| Integrated Devices Technolgy, Inc.
| IBIS Model Of 82P2821
| BH_640
[IBIS ver]	3.2
[File name]	82p2821.ibs
[File Rev]	1.0
[Date]		Aug. 15, 2005
[Source]	Integrated Devices Technolgy, Inc.
[Notes]   1. Temperatures: typ=25C, min=90C, max=-40C .
   2. simulator: hspice
   3. The IBIS models are validated with hspice models
[Disclaimer]	 Integrated Device Technology, Inc. ("IDT") hereby grants
		 the user of this IBIS model a non-exclusive, nontransferable
		 license to use this IBIS model under the following terms.
		 The user is granted this license only to use the IBIS model
		 and is not granted rights to sell, copy (except as needed to
		 run the IBIS model), rent, lease or sub-license the IBIS model
		 in whole or in part, or in modified form to anyone. The User
		 may modify the IBIS model to suit its specific applications,
		 but rights to derivative works and such modifications shall
		 belong to IDT. This IBIS model is provided on an AS IS" basis
		 and IDT makes absolutely no warranty with respect to the
		 information contained herein. IDT DISCLAIMS AND CUSTOMER WAIVES
		 ALL WARRANTIES, EXPRESS AND IMPLIED, INCLUDING WARRANTIES
		 OF MERCHANTABILITY AND FITNESS FOR A PARTICULAR PURPOSE. THE
		 ENTIRE RISK AS TO QUALITY AND PERFORMANCE IS WITH THE USER ACCORDINGLY,
		 IN NO EVENT SHALL IDT BE LIABLE FOR ANY DIRECT OR
		 INDIRECT DAMAGES, WHETHER IN CONTRACT OR TORT, INCLUDING ANY
		 LOST PROFITS OR OTHER INCIDENTAL, CONSEQUENTIAL, EXEMPLARY, OR
		 PUNITIVE DAMAGES ARISING OUT OF THE USE OR APPLICATION OF THE
		 IBIS model. Further, IDT reserves the right to make changes
		 without notice to
[Copyright]	Copyright 2005, Integrated Devices Technolgy, Inc.,
   All Rights Reserved.
|   Component 82P2821
[Component]	82P2821
[Manufacturer]	Integrated Devices Technolgy, Inc.
[Package]
| variable   typ   min   max
R_pkg   0.3500   0.2100   0.5700
L_pkg   7.3400nH   3.9900nH   14.3900nH
C_pkg   0.8400pF   0.2900pF   2.2800pF
[Pin]  signal_name   model_name   R_pin   L_pin   C_pin
AH15   A0   PITSN   0.28   5.98nH   0.54pF
AJ15   A1   PITSN   0.34   6.70nH   0.54pF
AK13   A10   PITSN   0.31   6.28nH   0.65pF
AK15   A2   PITSN   0.32   6.54nH   0.56pF
AG14   A3   PITSN   0.30   5.73nH   0.40pF
AH14   A4   PITSN   0.38   7.07nH   0.53pF
AJ14   A5   PITSN   0.41   7.66nH   0.54pF
AK14   A6   PITSN   0.38   7.05nH   0.46pF
AG13   A7   PITSN   0.31   5.66nH   0.45pF
AH13   A8   PITSN   0.29   5.36nH   0.81pF
AJ13   A9   PITSN   0.39   7.29nH   0.51pF
AG15   ALE_AS   PITSN   0.24   5.67nH   0.39pF
AH17   CLKA   PITSN   0.33   6.42nH   0.61pF
AG17   CLKB   PITSN   0.24   5.26nH   0.39pF
AG18   CLKE1   PTT04   0.29   5.36nH   0.59pF
AH18   CLKT1   PTT04   0.33   6.58nH   0.63pF
AJ17   CSB   PITSN   0.28   5.88nH   0.68pF
AG12   D0   PBRT16N   0.47   9.50nH   0.64pF
AH12   D1   PBRT16N   0.30   6.21nH   0.51pF
AJ12   D2   PBRT16N   0.42   8.14nH   0.52pF
AK12   D3   PBRT16N   0.39   7.39nH   0.54pF
AG11   D4   PBRT16N   0.44   8.75nH   0.72pF
AH11   D5   PBRT16N   0.39   7.82nH   0.57pF
AJ11   D6   PBRT16N   0.39   7.68nH   0.41pF
AK11   D7   PBRT16N   0.34   8.06nH   0.52pF
AF9   GPIO0   PBRT04N   0.34   7.73nH   0.90pF
AF10   GPIO1   PBRT04N   0.52   11.9nH   0.66pF
AF15   IM   PITSU   0.32   6.53nH   0.51pF
AF14   INT_MOTB   PITSU   0.24   5.64nH   0.42pF
AK16   INTB   PTT12   0.36   7.13nH   0.56pF
AF17   LLOS   PTT04   0.28   5.17nH   0.34pF
AF18   LLOS0   PTT04   0.46   9.61nH   1.07pF
AF19   MCKSEL0   PITSN   0.27   5.21nH   0.34pF
AF20   MCKSEL1   PITSN   0.23   5.15nH   0.49pF
AF21   MCKSEL2   PITSN   0.34   7.31nH   0.86pF
AF22   MCKSEL3   PITSN   0.32   6.54nH   0.83pF
AK19   MCLK   PITSN   0.39   7.91nH   0.46pF
AJ10   OE   PITSD   0.32   7.10nH   0.47pF
AG16   P_SB   PITSU   0.35   7.13nH   0.57pF
AK10   RCLK0   PTT04   0.39   7.36nH   0.29pF
AD2   RCLK1   PTT04   0.42   9.35nH   0.42pF
AG29   RCLK10   PTT04   0.35   6.26nH   0.74pF
A28   RCLK11   PTT04   0.41   8.24nH   0.48pF
C25   RCLK12   PTT04   0.39   7.20nH   0.78pF
A23   RCLK13   PTT04   0.45   8.79nH   0.79pF
A20   RCLK14   PTT04   0.40   9.11nH   0.77pF
C19   RCLK15   PTT04   0.46   9.65nH   0.80pF
A17   RCLK16   PTT04   0.41   8.42nH   0.86pF
C16   RCLK17   PTT04   0.47   10.0nH   0.96pF
B14   RCLK18   PTT04   0.39   8.51nH   0.74pF
D13   RCLK19   PTT04   0.42   8.85nH   0.82pF
AH2   RCLK2   PTT04   0.38   8.73nH   0.50pF
B11   RCLK20   PTT04   0.39   8.78nH   0.72pF
B8   RCLK21   PTT04   0.34   7.03nH   0.82pF
AK4   RCLK3   PTT04   0.52   11.3nH   0.74pF
AK7   RCLK4   PTT04   0.48   10.5nH   0.79pF
AH8   RCLK5   PTT04   0.42   9.12nH   0.69pF
AH20   RCLK6   PTT04   0.43   9.22nH   0.62pF
AK22   RCLK7   PTT04   0.37   7.90nH   0.40pF
AK25   RCLK8   PTT04   0.33   6.74nH   0.38pF
AH26   RCLK9   PTT04   0.39   8.02nH   0.48pF
AG9   RDN0   PTT04   0.33   7.35nH   1.00pF
AD1   RDN1   PTT04   0.44   10.0nH   0.35pF
AH30   RDN10   PTT04   0.32   6.26nH   0.69pF
B28   RDN11   PTT04   0.33   5.72nH   1.17pF
D25   RDN12   PTT04   0.37   7.17nH   1.04pF
B23   RDN13   PTT04   0.33   6.61nH   1.04pF
B20   RDN14   PTT04   0.45   9.93nH   0.77pF
D19   RDN15   PTT04   0.45   9.44nH   0.91pF
B17   RDN16   PTT04   0.39   7.99nH   0.84pF
A15   RDN17   PTT04   0.39   8.07nH   1.01pF
C14   RDN18   PTT04   0.39   8.31nH   0.79pF
A12   RDN19   PTT04   0.41   8.77nH   0.90pF
AH1   RDN2   PTT04   0.37   8.66nH   0.52pF
C11   RDN20   PTT04   0.33   6.93nH   0.79pF
C8   RDN21   PTT04   0.31   6.60nH   0.81pF
AG3   RDN3   PTT04   0.44   10.7nH   0.56pF
AG6   RDN4   PTT04   0.42   9.64nH   0.73pF
AJ8   RDN5   PTT04   0.41   8.75nH   0.96pF
AJ20   RDN6   PTT04   0.37   8.35nH   1.07pF
AG21   RDN7   PTT04   0.33   6.10nH   0.88pF
AG24   RDN8   PTT04   0.40   8.43nH   0.61pF
AJ26   RDN9   PTT04   0.26   6.07nH   0.61pF
AH9   RDP0   PTT04   0.42   7.91nH   0.60pF
AC4   RDP1   PTT04   0.38   8.20nH   0.46pF
AH29   RDP10   PTT04   0.40   7.55nH   0.60pF
A27   RDP11   PTT04   0.35   6.67nH   0.59pF
A24   RDP12   PTT04   0.43   8.13nH   0.57pF
C23   RDP13   PTT04   0.39   7.69nH   0.84pF
C20   RDP14   PTT04   0.43   9.57nH   0.74pF
A18   RDP15   PTT04   0.42   8.49nH   0.89pF
C17   RDP16   PTT04   0.37   7.62nH   0.89pF
B15   RDP17   PTT04   0.38   8.42nH   0.74pF
D14   RDP18   PTT04   0.31   6.60nH   0.71pF
B12   RDP19   PTT04   0.34   6.91nH   0.68pF
AG1   RDP2   PTT04   0.42   10.1nH   0.46pF
D11   RDP20   PTT04   0.31   6.61nH   0.75pF
D8   RDP21   PTT04   0.36   7.67nH   0.67pF
AH3   RDP3   PTT04   0.48   10.5nH   0.64pF
AH6   RDP4   PTT04   0.43   9.73nH   0.92pF
AK8   RDP5   PTT04   0.47   10.8nH   0.75pF
AK20   RDP6   PTT04   0.40   8.75nH   0.69pF
AH21   RDP7   PTT04   0.41   8.81nH   0.48pF
AH24   RDP8   PTT04   0.39   8.22nH   0.38pF
AK26   RDP9   PTT04   0.33   6.79nH   0.35pF
D29   REF   NC   0.48   10.1nH   2.28pF
AK18   REFA   PTT12   0.38   7.78nH   0.50pF
AJ18   REFB   PTT12   0.35   7.00nH   0.77pF
AH10   RIM   PITSD   0.39   7.91nH   0.60pF
N3   RRING0   NC   0.33   5.93nH   0.89pF
P5   RRING1   NC   0.29   4.96nH   1.02pF
R28   RRING10   NC   0.34   5.15nH   1.46pF
P26   RRING11   NC   0.28   3.99nH   1.14pF
K28   RRING12   NC   0.31   4.86nH   0.98pF
K26   RRING13   NC   0.28   4.37nH   0.83pF
F26   RRING14   NC   0.34   5.84nH   0.96pF
E28   RRING15   NC   0.28   4.50nH   0.88pF
E6   RRING16   NC   0.31   5.23nH   0.80pF
D5   RRING17   NC   0.36   6.36nH   0.88pF
E3   RRING18   NC   0.31   4.78nH   0.90pF
F4   RRING19   NC   0.34   5.47nH   0.97pF
U4   RRING2   NC   NA   NA   NA
G5   RRING20   NC   0.33   5.37nH   1.01pF
L5   RRING21   NC   0.36   6.62nH   1.08pF
V5   RRING3   NC   0.31   4.91nH   1.39pF
Y4   RRING4   NC   0.31   4.62nH   1.31pF
AA5   RRING5   NC   0.37   5.84nH   1.27pF
AD28   RRING6   NC   0.36   5.60nH   1.55pF
AD26   RRING7   NC   0.36   5.31nH   1.79pF
Y26   RRING8   NC   0.42   7.23nH   1.70pF
W27   RRING9   NC   0.36   5.61nH   1.65pF
AG10   RSTB   PITSU   0.44   8.98nH   0.58pF
P3   RTIP0   NC   0.34   5.85nH   1.07pF
R5   RTIP1   NC   0.29   4.71nH   1.01pF
T28   RTIP10   NC   0.32   5.36nH   1.01pF
R26   RTIP11   NC   0.28   4.49nH   1.07pF
L28   RTIP12   NC   0.33   5.51nH   1.00pF
L26   RTIP13   NC   0.28   4.48nH   0.87pF
G26   RTIP14   NC   0.33   5.53nH   0.90pF
F28   RTIP15   NC   0.26   4.23nH   0.98pF
D6   RTIP16   NC   0.31   5.22nH   0.85pF
D4   RTIP17   NC   0.37   6.05nH   1.01pF
D3   RTIP18   NC   0.30   4.59nH   0.91pF
G4   RTIP19   NC   0.34   5.34nH   1.04pF
V4   RTIP2   NC   NA   NA   NA
H5   RTIP20   NC   0.33   5.34nH   1.02pF
M5   RTIP21   NC   0.36   7.71nH   1.14pF
W5   RTIP3   NC   0.32   5.32nH   0.98pF
AA4   RTIP4   NC   0.29   5.19nH   0.98pF
AB5   RTIP5   NC   0.34   6.41nH   0.78pF
AE28   RTIP6   NC   0.34   5.96nH   0.93pF
AE26   RTIP7   NC   0.34   5.60nH   1.05pF
AA26   RTIP8   NC   0.41   7.32nH   1.18pF
W28   RTIP9   NC   0.34   5.84nH   1.04pF
AK17   SCLK_DSB_RDB   PITSN   0.38   7.68nH   0.45pF
AH16   SDI_RWB_WRB   PITSN   0.32   6.44nH   0.82pF
AJ16   SDO_RDY_ACKB   PTT12   0.40   8.36nH   0.51pF
AF6   TCK   PITSN   0.34   8.72nH   0.69pF
AJ9   TCLK0   PITSN   0.32   7.10nH   0.50pF
AC3   TCLK1   PITSN   0.39   8.95nH   0.44pF
AG28   TCLK10   PITSN   0.29   6.20nH   0.61pF
B27   TCLK11   PITSN   0.34   6.93nH   0.79pF
B24   TCLK12   PITSN   0.40   7.18nH   0.70pF
D23   TCLK13   PITSN   0.42   8.16nH   1.07pF
D20   TCLK14   PITSN   0.41   8.00nH   0.89pF
B18   TCLK15   PITSN   0.40   8.16nH   0.89pF
D17   TCLK16   PITSN   0.36   7.44nH   0.92pF
C15   TCLK17   PITSN   0.38   7.75nH   0.78pF
A13   TCLK18   PITSN   0.32   6.75nH   0.84pF
C12   TCLK19   PITSN   0.32   6.83nH   0.75pF
AF3   TCLK2   PITSN   0.40   9.68nH   0.40pF
A10   TCLK20   PITSN   0.29   6.20nH   0.77pF
A7   TCLK21   PITSN   0.33   7.11nH   0.71pF
AJ3   TCLK3   PITSN   0.39   9.12nH   0.53pF
AJ6   TCLK4   PITSN   0.45   10.0nH   1.13pF
AG7   TCLK5   PITSN   0.40   9.80nH   0.42pF
AG19   TCLK6   PITSN   0.42   10.7nH   0.88pF
AJ21   TCLK7   PITSN   0.35   8.10nH   1.00pF
AJ24   TCLK8   PITSN   0.35   7.07nH   0.69pF
AG25   TCLK9   PITSN   0.33   7.99nH   0.55pF
AF5   TDI   PITSU   0.52   13.0nH   0.93pF
AK9   TDN0   PBRT04N   0.43   8.12nH   0.46pF
AC2   TDN1   PBRT04N   0.40   9.19nH   0.54pF
AH28   TDN10   PBRT04N   0.34   6.49nH   0.72pF
C27   TDN11   PBRT04N   0.40   7.67nH   0.56pF
C24   TDN12   PBRT04N   0.41   8.39nH   0.65pF
A22   TDN13   PBRT04N   0.43   8.04nH   0.84pF
A19   TDN14   PBRT04N   0.39   7.69nH   0.87pF
C18   TDN15   PBRT04N   0.38   8.03nH   0.98pF
A16   TDN16   PBRT04N   0.45   9.75nH   0.81pF
D15   TDN17   PBRT04N   0.35   7.12nH   0.83pF
B13   TDN18   PBRT04N   0.37   7.89nH   0.76pF
D12   TDN19   PBRT04N   0.32   6.71nH   0.70pF
AF2   TDN2   PBRT04N   0.37   8.52nH   0.35pF
B10   TDN20   PBRT04N   0.35   7.58nH   0.77pF
B7   TDN21   PBRT04N   0.30   6.22nH   0.73pF
AK3   TDN3   PBRT04N   0.45   10.0nH   0.74pF
AK6   TDN4   PBRT04N   0.51   11.7nH   1.07pF
AH7   TDN5   PBRT04N   0.44   9.72nH   0.81pF
AH19   TDN6   PBRT04N   0.46   10.2nH   0.68pF
AK21   TDN7   PBRT04N   0.38   7.55nH   0.76pF
AK24   TDN8   PBRT04N   0.34   6.66nH   0.45pF
AH25   TDN9   PBRT04N   0.38   8.44nH   0.31pF
AF7   TDO   PTT12   0.56   12.9nH   0.93pF
AG8   TDP0   PITSN   0.40   7.67nH   0.54pF
AC1   TDP1   PITSN   0.44   10.2nH   0.42pF
AJ28   TDP10   PITSN   0.30   7.08nH   0.56pF
D27   TDP11   PITSN   0.32   6.06nH   0.71pF
D24   TDP12   PITSN   0.40   7.64nH   0.93pF
B22   TDP13   PITSN   0.36   7.25nH   1.17pF
B19   TDP14   PITSN   0.41   8.09nH   0.78pF
D18   TDP15   PITSN   0.34   7.27nH   1.08pF
B16   TDP16   PITSN   0.44   9.24nH   0.92pF
A14   TDP17   PITSN   0.31   5.97nH   0.94pF
C13   TDP18   PITSN   0.35   7.44nH   0.86pF
A11   TDP19   PITSN   0.29   5.96nH   0.81pF
AF1   TDP2   PITSN   0.37   7.69nH   0.81pF
C10   TDP20   PITSN   0.38   7.88nH   0.74pF
C7   TDP21   PITSN   0.27   5.58nH   0.78pF
AG2   TDP3   PITSN   0.44   10.3nH   0.52pF
AG5   TDP4   PITSN   0.48   10.0nH   0.96pF
AJ7   TDP5   PITSN   0.46   9.38nH   1.04pF
AJ19   TDP6   PITSN   0.40   11.5nH   0.41pF
AG20   TDP7   PITSN   0.41   8.25nH   0.80pF
AG23   TDP8   PITSN   0.37   7.13nH   0.57pF
AJ25   TDP9   PITSN   0.25   5.85nH   0.51pF
AF12   TEHW   PITSU   0.57   11.8nH   0.81pF
AF11   TEHWE   PITSU   0.26   6.45nH   0.59pF
AF13   TESTSE   PITSD   0.21   5.04nH   0.31pF
AE5   TMS   PITSU   0.36   9.52nH   0.96pF
K1   TRING0   NC   0.33   6.90nH   1.22pF
M2   TRING1   NC   0.32   6.98nH   1.27pF
R30   TRING10   NC   0.28   6.00nH   1.14pF
N30   TRING11   NC   0.27   6.26nH   1.15pF
K30   TRING12   NC   0.29   6.31nH   1.03pF
H30   TRING13   NC   0.25   5.63nH   1.12pF
E30   TRING14   NC   0.27   5.74nH   1.10pF
C30   TRING15   NC   0.29   6.03nH   0.97pF
A6   TRING16   NC   0.23   4.96nH   1.13pF
B4   TRING17   NC   0.30   6.70nH   1.07pF
B3   TRING18   NC   0.31   6.78nH   1.09pF
D1   TRING19   NC   0.29   6.48nH   1.13pF
R2   TRING2   NC   NA   NA   NA
E1   TRING20   NC   0.33   7.13nH   1.19pF
J2   TRING21   NC   0.39   8.38nH   1.33pF
T1   TRING3   NC   0.33   6.86nH   1.27pF
W1   TRING4   NC   NA   NA   NA
AA2   TRING5   NC   0.34   6.94nH   1.15pF
AE30   TRING6   NC   0.33   6.82nH   1.15pF
AC30   TRING7   NC   0.34   7.53nH   1.31pF
Y30   TRING8   NC   0.33   7.09nH   1.22pF
V30   TRING9   NC   0.32   7.19nH   1.10pF
AF4   TRSTB   PITSD   0.55   14.3nH   0.68pF
L1   TTIP0   NC   0.33   7.57nH   0.85pF
M1   TTIP1   NC   0.32   7.45nH   0.87pF
T30   TTIP10   NC   0.30   7.37nH   0.85pF
P30   TTIP11   NC   0.27   6.49nH   0.93pF
L30   TTIP12   NC   0.29   6.73nH   0.83pF
J30   TTIP13   NC   0.26   6.13nH   0.85pF
F30   TTIP14   NC   0.27   6.21nH   0.72pF
D30   TTIP15   NC   0.29   6.55nH   0.68pF
A5   TTIP16   NC   0.25   5.85nH   0.93pF
A4   TTIP17   NC   0.31   7.07nH   0.83pF
A3   TTIP18   NC   0.31   7.38nH   0.77pF
C1   TTIP19   NC   0.32   7.72nH   0.77pF
R1   TTIP2   NC   NA   NA   NA
F1   TTIP20   NC   0.33   7.35nH   0.84pF
J1   TTIP21   NC   0.39   8.79nH   1.04pF
U1   TTIP3   NC   0.33   7.94nH   0.83pF
Y1   TTIP4   NC   NA   NA   NA
AA1   TTIP5   NC   0.34   6.96nH   0.78pF
AF30   TTIP6   NC   0.31   6.97nH   0.81pF
AD30   TTIP7   NC   0.33   7.61nH   0.68pF
AA30   TTIP8   NC   0.33   8.08nH   0.82pF
W30   TTIP9   NC   0.30   8.92nH   0.85pF
R4   VCOM0   NC   NA   NA   NA
P28   VCOM1   NC   NA   NA   NA
AF26   VDDIO   NC   0.32   5.83nH   0.72pF
N4   VDDR0   POWER   0.28   5.72nH   1.13pF
N5   VDDR1   POWER   0.27   5.67nH   1.17pF
T27   VDDR10   POWER   0.35   6.57nH   1.27pF
R27   VDDR11   POWER   0.33   6.90nH   1.17pF
N26   VDDR12   POWER   0.28   5.41nH   1.09pF
G27   VDDR13   POWER   0.24   4.55nH   0.96pF
E26   VDDR14   POWER   0.25   4.75nH   1.03pF
E27   VDDR15   POWER   0.25   5.62nH   0.98pF
E5   VDDR16   POWER   0.26   5.08nH   1.01pF
E4   VDDR17   POWER   0.22   4.83nH   0.86pF
F3   VDDR18   POWER   0.39   8.48nH   1.23pF
F5   VDDR19   POWER   0.36   7.20nH   1.22pF
T5   VDDR2   POWER   0.30   6.43nH   1.44pF
G3   VDDR20   POWER   0.34   6.37nH   1.33pF
H3   VDDR21   POWER   0.35   6.89nH   1.32pF
U5   VDDR3   POWER   0.25   5.41nH   1.04pF
AB4   VDDR4   POWER   0.26   5.25nH   1.10pF
AC5   VDDR5   POWER   0.30   6.05nH   1.07pF
AF28   VDDR6   POWER   0.30   5.79nH   0.94pF
AF27   VDDR7   POWER   0.26   5.25nH   0.77pF
AD27   VDDR8   POWER   0.42   8.13nH   1.27pF
U27   VDDR9   POWER   0.35   6.21nH   1.17pF
K2   VDDT0   POWER   0.36   8.85nH   1.14pF
L2   VDDT1   POWER   0.35   8.69nH   1.37pF
R29   VDDT10   POWER   0.24   5.61nH   1.02pF
P29   VDDT11   POWER   0.23   5.49nH   1.11pF
K29   VDDT12   POWER   0.23   5.58nH   1.02pF
J29   VDDT13   POWER   0.30   7.45nH   1.00pF
F29   VDDT14   POWER   0.31   7.79nH   0.95pF
E29   VDDT15   POWER   0.23   5.36nH   0.95pF
C6   VDDT16   POWER   0.28   6.64nH   1.18pF
C4   VDDT17   POWER   0.25   6.08nH   1.09pF
C3   VDDT18   POWER   0.26   6.36nH   1.06pF
C2   VDDT19   POWER   0.36   9.25nH   1.15pF
P2   VDDT2   POWER   NA   NA   NA
F2   VDDT20   POWER   0.29   6.08nH   1.17pF
H2   VDDT21   POWER   0.31   6.83nH   1.20pF
R3   VDDT3   POWER   0.36   8.87nH   1.16pF
W2   VDDT4   POWER   0.37   8.79nH   1.68pF
Y2   VDDT5   POWER   0.39   9.04nH   1.06pF
AF29   VDDT6   POWER   0.37   8.47nH   1.01pF
AC29   VDDT7   POWER   0.37   9.28nH   0.72pF
AA29   VDDT8   POWER   0.28   7.67nH   1.02pF
Y29   VDDT9   POWER   0.37   9.13nH   1.15pF
F10   GNDD   GND   NA   NA   NA
F11   GNDD   GND   NA   NA   NA
F12   GNDD   GND   NA   NA   NA
F13   GNDD   GND   NA   NA   NA
F14   GNDD   GND   NA   NA   NA
F15   GNDD   GND   NA   NA   NA
F16   GNDD   GND   NA   NA   NA
F17   GNDD   GND   NA   NA   NA
F18   GNDD   GND   NA   NA   NA
F19   GNDD   GND   NA   NA   NA
F20   GNDD   GND   NA   NA   NA
F21   GNDD   GND   NA   NA   NA
F22   GNDD   GND   NA   NA   NA
F23   GNDD   GND   NA   NA   NA
F24   GNDD   GND   NA   NA   NA
M12   GNDD   GND   NA   NA   NA
M13   GNDD   GND   NA   NA   NA
M14   GNDD   GND   NA   NA   NA
M15   GNDD   GND   NA   NA   NA
M16   GNDD   GND   NA   NA   NA
M17   GNDD   GND   NA   NA   NA
M18   GNDD   GND   NA   NA   NA
M19   GNDD   GND   NA   NA   NA
N12   GNDD   GND   NA   NA   NA
N13   GNDD   GND   NA   NA   NA
N14   GNDD   GND   NA   NA   NA
N15   GNDD   GND   NA   NA   NA
N16   GNDD   GND   NA   NA   NA
N17   GNDD   GND   NA   NA   NA
N18   GNDD   GND   NA   NA   NA
N19   GNDD   GND   NA   NA   NA
P12   GNDD   GND   NA   NA   NA
P13   GNDD   GND   NA   NA   NA
P14   GNDD   GND   NA   NA   NA
P15   GNDD   GND   NA   NA   NA
P16   GNDD   GND   NA   NA   NA
P17   GNDD   GND   NA   NA   NA
P18   GNDD   GND   NA   NA   NA
P19   GNDD   GND   NA   NA   NA
R12   GNDD   GND   NA   NA   NA
R13   GNDD   GND   NA   NA   NA
R14   GNDD   GND   NA   NA   NA
R15   GNDD   GND   NA   NA   NA
R16   GNDD   GND   NA   NA   NA
R17   GNDD   GND   NA   NA   NA
R18   GNDD   GND   NA   NA   NA
R19   GNDD   GND   NA   NA   NA
T12   GNDD   GND   NA   NA   NA
T13   GNDD   GND   NA   NA   NA
T14   GNDD   GND   NA   NA   NA
T15   GNDD   GND   NA   NA   NA
T16   GNDD   GND   NA   NA   NA
T17   GNDD   GND   NA   NA   NA
T18   GNDD   GND   NA   NA   NA
T19   GNDD   GND   NA   NA   NA
U12   GNDD   GND   NA   NA   NA
U13   GNDD   GND   NA   NA   NA
U14   GNDD   GND   NA   NA   NA
U15   GNDD   GND   NA   NA   NA
U16   GNDD   GND   NA   NA   NA
U17   GNDD   GND   NA   NA   NA
U18   GNDD   GND   NA   NA   NA
U19   GNDD   GND   NA   NA   NA
V12   GNDD   GND   NA   NA   NA
V13   GNDD   GND   NA   NA   NA
V14   GNDD   GND   NA   NA   NA
V15   GNDD   GND   NA   NA   NA
V16   GNDD   GND   NA   NA   NA
V17   GNDD   GND   NA   NA   NA
V18   GNDD   GND   NA   NA   NA
V19   GNDD   GND   NA   NA   NA
W12   GNDD   GND   NA   NA   NA
W13   GNDD   GND   NA   NA   NA
W14   GNDD   GND   NA   NA   NA
W15   GNDD   GND   NA   NA   NA
W16   GNDD   GND   NA   NA   NA
W17   GNDD   GND   NA   NA   NA
W18   GNDD   GND   NA   NA   NA
W19   GNDD   GND   NA   NA   NA
AE7   GNDD   GND   NA   NA   NA
AE8   GNDD   GND   NA   NA   NA
AE12   GNDD   GND   NA   NA   NA
AE13   GNDD   GND   NA   NA   NA
AF23   GNDD   GND   NA   NA   NA
AF24   GNDD   GND   NA   NA   NA
A1   GNDA   GND   NA   NA   NA
A29   GNDA   GND   NA   NA   NA
A30   GNDA   GND   NA   NA   NA
B1   GNDA   GND   NA   NA   NA
B29   GNDA   GND   NA   NA   NA
B30   GNDA   GND   NA   NA   NA
F6   GNDA   GND   NA   NA   NA
F7   GNDA   GND   NA   NA   NA
F8   GNDA   GND   NA   NA   NA
F25   GNDA   GND   NA   NA   NA
G6   GNDA   GND   NA   NA   NA
G25   GNDA   GND   NA   NA   NA
H6   GNDA   GND   NA   NA   NA
H25   GNDA   GND   NA   NA   NA
J6   GNDA   GND   NA   NA   NA
J25   GNDA   GND   NA   NA   NA
K6   GNDA   GND   NA   NA   NA
K25   GNDA   GND   NA   NA   NA
L6   GNDA   GND   NA   NA   NA
L25   GNDA   GND   NA   NA   NA
M6   GNDA   GND   NA   NA   NA
M25   GNDA   GND   NA   NA   NA
N6   GNDA   GND   NA   NA   NA
N25   GNDA   GND   NA   NA   NA
P6   GNDA   GND   NA   NA   NA
P25   GNDA   GND   NA   NA   NA
R6   GNDA   GND   NA   NA   NA
R25   GNDA   GND   NA   NA   NA
T6   GNDA   GND   NA   NA   NA
T25   GNDA   GND   NA   NA   NA
U6   GNDA   GND   NA   NA   NA
U25   GNDA   GND   NA   NA   NA
V6   GNDA   GND   NA   NA   NA
V25   GNDA   GND   NA   NA   NA
W6   GNDA   GND   NA   NA   NA
W25   GNDA   GND   NA   NA   NA
W26   GNDA   GND   NA   NA   NA
Y6   GNDA   GND   NA   NA   NA
Y25   GNDA   GND   NA   NA   NA
AA6   GNDA   GND   NA   NA   NA
AA25   GNDA   GND   NA   NA   NA
AB1   GNDA   GND   NA   NA   NA
AB6   GNDA   GND   NA   NA   NA
AB25   GNDA   GND   NA   NA   NA
AB26   GNDA   GND   NA   NA   NA
AC6   GNDA   GND   NA   NA   NA
AC25   GNDA   GND   NA   NA   NA
AC26   GNDA   GND   NA   NA   NA
AD6   GNDA   GND   NA   NA   NA
AD25   GNDA   GND   NA   NA   NA
AE6   GNDA   GND   NA   NA   NA
AE25   GNDA   GND   NA   NA   NA
AJ1   GNDA   GND   NA   NA   NA
AJ29   GNDA   GND   NA   NA   NA
AJ30   GNDA   GND   NA   NA   NA
AK1   GNDA   GND   NA   NA   NA
AK29   GNDA   GND   NA   NA   NA
AK30   GNDA   GND   NA   NA   NA
B5   GNDT   GND   NA   NA   NA
B6   GNDT   GND   NA   NA   NA
C5   GNDT   GND   NA   NA   NA
D2   GNDT   GND   NA   NA   NA
D28   GNDT   GND   NA   NA   NA
E2   GNDT   GND   NA   NA   NA
H28   GNDT   GND   NA   NA   NA
H29   GNDT   GND   NA   NA   NA
J3   GNDT   GND   NA   NA   NA
J5   GNDT   GND   NA   NA   NA
J28   GNDT   GND   NA   NA   NA
K3   GNDT   GND   NA   NA   NA
K5   GNDT   GND   NA   NA   NA
L3   GNDT   GND   NA   NA   NA
M3   GNDT   GND   NA   NA   NA
M28   GNDT   GND   NA   NA   NA
N28   GNDT   GND   NA   NA   NA
N29   GNDT   GND   NA   NA   NA
T2   GNDT   GND   NA   NA   NA
U2   GNDT   GND   NA   NA   NA
U28   GNDT   GND   NA   NA   NA
V28   GNDT   GND   NA   NA   NA
V29   GNDT   GND   NA   NA   NA
W29   GNDT   GND   NA   NA   NA
AA3   GNDT   GND   NA   NA   NA
AB2   GNDT   GND   NA   NA   NA
AB28   GNDT   GND   NA   NA   NA
AD29   GNDT   GND   NA   NA   NA
AE29   GNDT   GND   NA   NA   NA
A2   VDDA   POWER   NA   NA   NA
B2   VDDA   POWER   NA   NA   NA
J26   VDDA   POWER   NA   NA   NA
K27   VDDA   POWER   NA   NA   NA
L4   VDDA   POWER   NA   NA   NA
L27   VDDA   POWER   NA   NA   NA
M4   VDDA   POWER   NA   NA   NA
M26   VDDA   POWER   NA   NA   NA
T4   VDDA   POWER   NA   NA   NA
W4   VDDA   POWER   NA   NA   NA
Y5   VDDA   POWER   NA   NA   NA
Y27   VDDA   POWER   NA   NA   NA
Y28   VDDA   POWER   NA   NA   NA
AA27   VDDA   POWER   NA   NA   NA
AA28   VDDA   POWER   NA   NA   NA
AD5   VDDA   POWER   NA   NA   NA
AJ2   VDDA   POWER   NA   NA   NA
AK2   VDDA   POWER   NA   NA   NA
E7   VDDIO   POWER   NA   NA   NA
E8   VDDIO   POWER   NA   NA   NA
E10   VDDIO   POWER   NA   NA   NA
E11   VDDIO   POWER   NA   NA   NA
E12   VDDIO   POWER   NA   NA   NA
E21   VDDIO   POWER   NA   NA   NA
E22   VDDIO   POWER   NA   NA   NA
E23   VDDIO   POWER   NA   NA   NA
E24   VDDIO   POWER   NA   NA   NA
E25   VDDIO   POWER   NA   NA   NA
AE9   VDDIO   POWER   NA   NA   NA
AE10   VDDIO   POWER   NA   NA   NA
AE15   VDDIO   POWER   NA   NA   NA
AE16   VDDIO   POWER   NA   NA   NA
AE17   VDDIO   POWER   NA   NA   NA
AE18   VDDIO   POWER   NA   NA   NA
AE22   VDDIO   POWER   NA   NA   NA
AE23   VDDIO   POWER   NA   NA   NA
AE24   VDDIO   POWER   NA   NA   NA
E14   VDDD   POWER   NA   NA   NA
E15   VDDD   POWER   NA   NA   NA
E16   VDDD   POWER   NA   NA   NA
E17   VDDD   POWER   NA   NA   NA
E18   VDDD   POWER   NA   NA   NA
E19   VDDD   POWER   NA   NA   NA
AE11   VDDD   POWER   NA   NA   NA
AE14   VDDD   POWER   NA   NA   NA
AE19   VDDD   POWER   NA   NA   NA
AE20   VDDD   POWER   NA   NA   NA
AE21   VDDD   POWER   NA   NA   NA
A8   NC   NC   NA   NA   NA
A9   NC   NC   NA   NA   NA
A21   NC   NC   NA   NA   NA
A25   NC   NC   NA   NA   NA
A26   NC   NC   NA   NA   NA
B9   NC   NC   NA   NA   NA
B21   NC   NC   NA   NA   NA
B25   NC   NC   NA   NA   NA
B26   NC   NC   NA   NA   NA
C9   NC   NC   NA   NA   NA
C21   NC   NC   NA   NA   NA
C22   NC   NC   NA   NA   NA
C26   NC   NC   NA   NA   NA
C28   NC   NC   NA   NA   NA
C29   NC   NC   NA   NA   NA
D7   NC   NC   NA   NA   NA
D9   NC   NC   NA   NA   NA
D10   NC   NC   NA   NA   NA
D16   NC   NC   NA   NA   NA
D21   NC   NC   NA   NA   NA
D22   NC   NC   NA   NA   NA
D26   NC   NC   NA   NA   NA
E9   NC   NC   NA   NA   NA
E13   NC   NC   NA   NA   NA
E20   NC   NC   NA   NA   NA
F9   NC   NC   NA   NA   NA
F27   NC   NC   NA   NA   NA
G1   NC   NC   NA   NA   NA
G2   NC   NC   NA   NA   NA
G28   NC   NC   NA   NA   NA
G29   NC   NC   NA   NA   NA
G30   NC   NC   NA   NA   NA
H1   NC   NC   NA   NA   NA
H4   NC   NC   NA   NA   NA
H26   NC   NC   NA   NA   NA
H27   NC   NC   NA   NA   NA
J4   NC   NC   NA   NA   NA
J27   NC   NC   NA   NA   NA
K4   NC   NC   NA   NA   NA
L29   NC   NC   NA   NA   NA
M27   NC   NC   NA   NA   NA
M29   NC   NC   NA   NA   NA
M30   NC   NC   NA   NA   NA
N1   NC   NC   NA   NA   NA
N2   NC   NC   NA   NA   NA
N27   NC   NC   NA   NA   NA
P1   NC   NC   NA   NA   NA
P4   NC   NC   NA   NA   NA
P27   NC   NC   NA   NA   NA
T3   NC   NC   NA   NA   NA
T26   NC   NC   NA   NA   NA
T29   NC   NC   NA   NA   NA
U3   NC   NC   NA   NA   NA
U26   NC   NC   NA   NA   NA
U29   NC   NC   NA   NA   NA
U30   NC   NC   NA   NA   NA
V1   NC   NC   NA   NA   NA
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| Models and submodels in the file (7): PBRT04N (I/O), PBRT16N (I/O), PITSD (Input), PITSN (Input), PITSU (Input), PTT04 (3-state), PTT12 (3-state)
